FUNCTION "Posizioni Linea" : VOID
TITLE =Gestione posizioni linea pallet
AUTHOR : MassimoZ
FAMILY : NovaSrl
VERSION : 0.1

BEGIN
NETWORK
TITLE ========= Posizioni Zona Accatastatrice 1 =======

NETWORK
TITLE =Pos Fermo pallet indietro *Zona Acc.1*
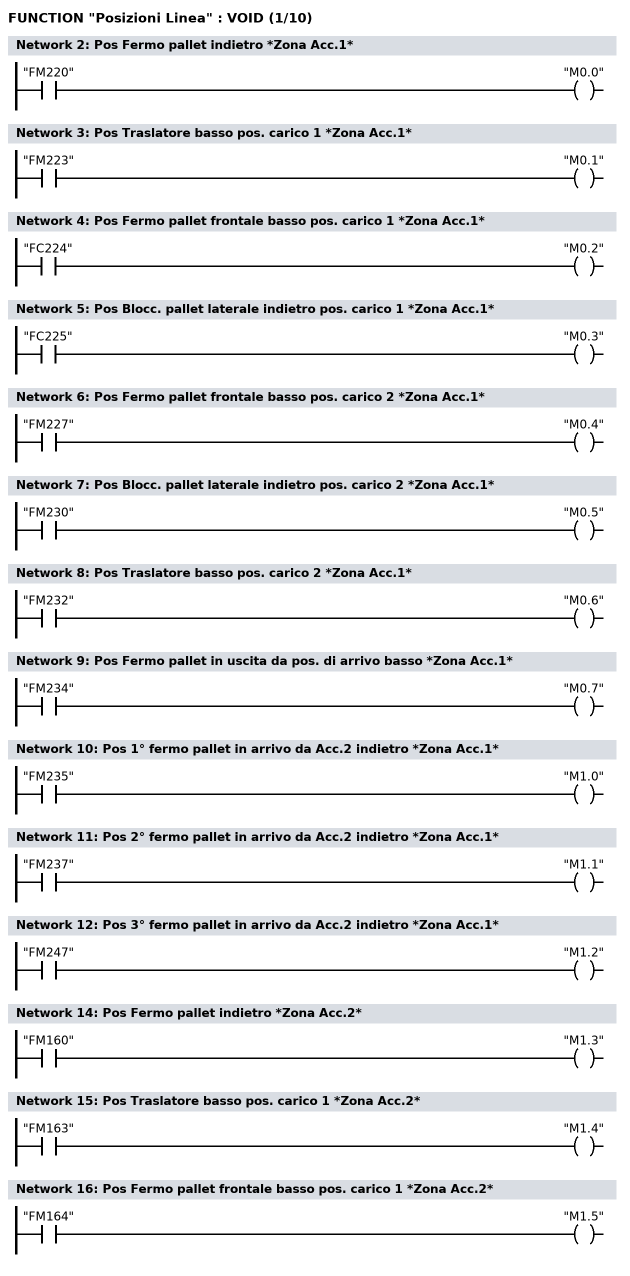
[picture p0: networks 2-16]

      U     "FM220";
      =     "M0.0";
NETWORK
TITLE =Pos Traslatore basso pos. carico 1 *Zona Acc.1*

      U     "FM223";
      =     "M0.1";
NETWORK
TITLE =Pos Fermo pallet frontale basso pos. carico 1 *Zona Acc.1*

      U     "FC224";
      =     "M0.2";
NETWORK
TITLE =Pos Blocc. pallet laterale indietro pos. carico 1 *Zona Acc.1*

      U     "FC225";
      =     "M0.3";
NETWORK
TITLE =Pos Fermo pallet frontale basso pos. carico 2 *Zona Acc.1*

      U     "FM227";
      =     "M0.4";
NETWORK
TITLE =Pos Blocc. pallet laterale indietro pos. carico 2 *Zona Acc.1*

      U     "FM230";
      =     "M0.5";
NETWORK
TITLE =Pos Traslatore basso pos. carico 2 *Zona Acc.1*

      U     "FM232";
      =     "M0.6";
NETWORK
TITLE =Pos Fermo pallet in uscita da pos. di arrivo basso *Zona Acc.1*

      U     "FM234";
      =     "M0.7";
NETWORK
TITLE =Pos 1° fermo pallet in arrivo da Acc.2 indietro *Zona Acc.1*

      U     "FM235";
      =     "M1.0";
NETWORK
TITLE =Pos 2° fermo pallet in arrivo da Acc.2 indietro *Zona Acc.1*

      U     "FM237";
      =     "M1.1";
NETWORK
TITLE =Pos 3° fermo pallet in arrivo da Acc.2 indietro *Zona Acc.1*

      U     "FM247";
      =     "M1.2";
NETWORK
TITLE ========= Posizioni Zona Accatastatrice 2 =======

NETWORK
TITLE =Pos Fermo pallet indietro *Zona Acc.2*

      U     "FM160";
      =     "M1.3";
NETWORK
TITLE =Pos Traslatore basso pos. carico 1 *Zona Acc.2*

      U     "FM163";
      =     "M1.4";
NETWORK
TITLE =Pos Fermo pallet frontale basso pos. carico 1 *Zona Acc.2*

      U     "FM164";
      =     "M1.5";
NETWORK
TITLE =Pos Blocc. pallet laterale indietro pos. carico 1 *Zona Acc.2*
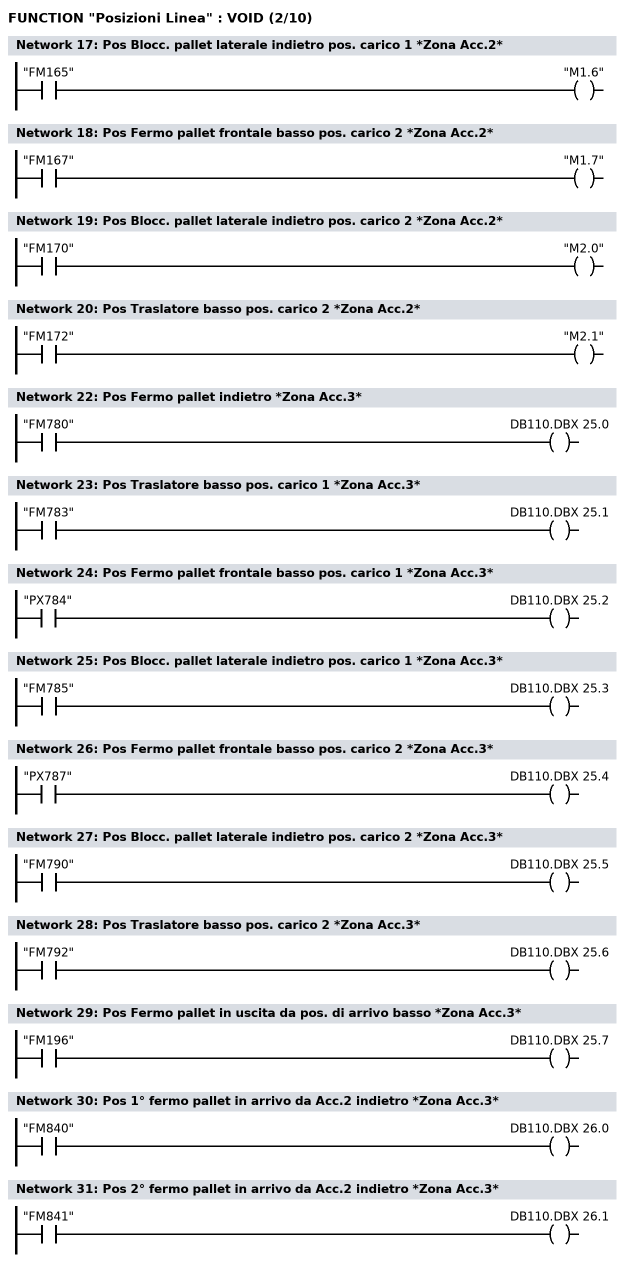
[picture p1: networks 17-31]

      U     "FM165";
      =     "M1.6";
NETWORK
TITLE =Pos Fermo pallet frontale basso pos. carico 2 *Zona Acc.2*

      U     "FM167";
      =     "M1.7";
NETWORK
TITLE =Pos Blocc. pallet laterale indietro pos. carico 2 *Zona Acc.2*

      U     "FM170";
      =     "M2.0";
NETWORK
TITLE =Pos Traslatore basso pos. carico 2 *Zona Acc.2*

      U     "FM172";
      =     "M2.1";
NETWORK
TITLE ========= Posizioni Zona Accatastatrice 3 =======

NETWORK
TITLE =Pos Fermo pallet indietro *Zona Acc.3*

      U     "FM780";
      =     DB110.DBX   25.0;
NETWORK
TITLE =Pos Traslatore basso pos. carico 1 *Zona Acc.3*

      U     "FM783";
      =     DB110.DBX   25.1;
NETWORK
TITLE =Pos Fermo pallet frontale basso pos. carico 1 *Zona Acc.3*

      U     "PX784";
      =     DB110.DBX   25.2;
NETWORK
TITLE =Pos Blocc. pallet laterale indietro pos. carico 1 *Zona Acc.3*

      U     "FM785";
      =     DB110.DBX   25.3;
NETWORK
TITLE =Pos Fermo pallet frontale basso pos. carico 2 *Zona Acc.3*

      U     "PX787";
      =     DB110.DBX   25.4;
NETWORK
TITLE =Pos Blocc. pallet laterale indietro pos. carico 2 *Zona Acc.3*

      U     "FM790";
      =     DB110.DBX   25.5;
NETWORK
TITLE =Pos Traslatore basso pos. carico 2 *Zona Acc.3*

      U     "FM792";
      =     DB110.DBX   25.6;
NETWORK
TITLE =Pos Fermo pallet in uscita da pos. di arrivo basso *Zona Acc.3*

      U     "FM196";
      =     DB110.DBX   25.7;
NETWORK
TITLE =Pos 1° fermo pallet in arrivo da Acc.2 indietro *Zona Acc.3*

      U     "FM840";
      =     DB110.DBX   26.0;
NETWORK
TITLE =Pos 2° fermo pallet in arrivo da Acc.2 indietro *Zona Acc.3*

      U     "FM841";
      =     DB110.DBX   26.1;
NETWORK
TITLE ======== Posizioni Zona Allineamento Bandiere =======

NETWORK
TITLE =Pos Allineamento bandiere alto *Zona Allineamento Bandiere*
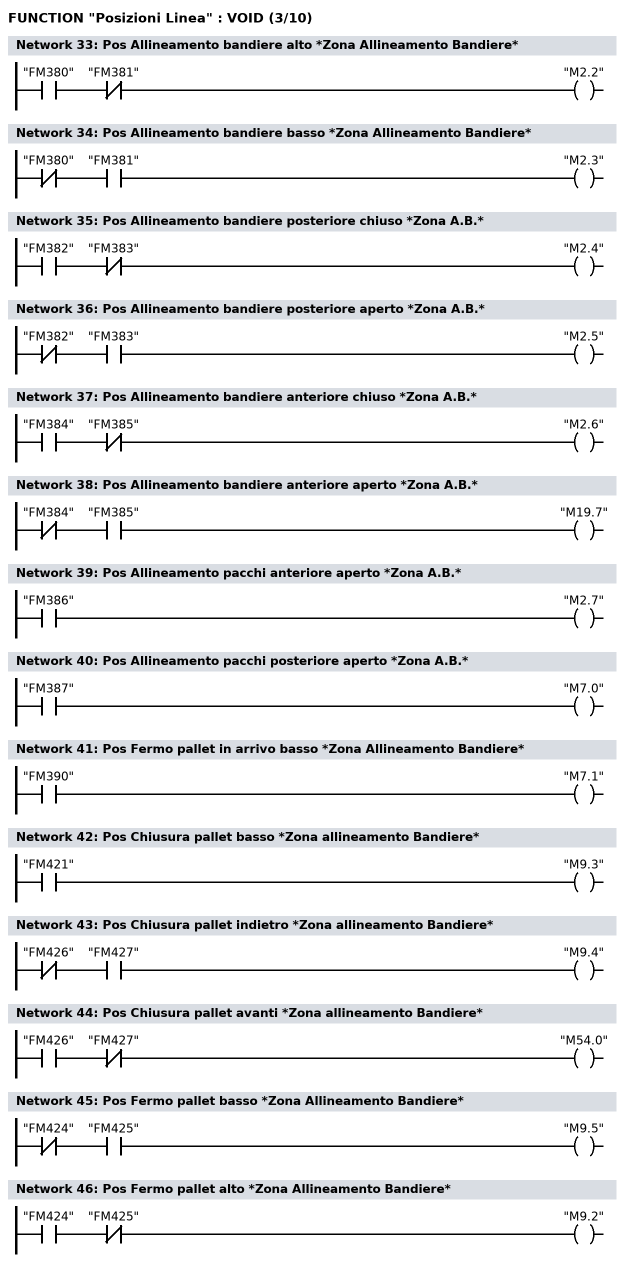
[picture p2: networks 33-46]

      U     "FM380";
      UN    "FM381";
      =     "M2.2";
NETWORK
TITLE =Pos Allineamento bandiere basso *Zona Allineamento Bandiere*

      UN    "FM380";
      U     "FM381";
      =     "M2.3";
NETWORK
TITLE =Pos Allineamento bandiere posteriore chiuso *Zona A.B.*

      U     "FM382";
      UN    "FM383";
      =     "M2.4";
NETWORK
TITLE =Pos Allineamento bandiere posteriore aperto *Zona A.B.*

      UN    "FM382";
      U     "FM383";
      =     "M2.5";
NETWORK
TITLE =Pos Allineamento bandiere anteriore chiuso *Zona A.B.*

      U     "FM384";
      UN    "FM385";
      =     "M2.6";
NETWORK
TITLE =Pos Allineamento bandiere anteriore aperto *Zona A.B.*

      UN    "FM384";
      U     "FM385";
      =     "M19.7";
NETWORK
TITLE =Pos Allineamento pacchi anteriore aperto *Zona A.B.*

      U     "FM386";
      =     "M2.7";
NETWORK
TITLE =Pos Allineamento pacchi posteriore aperto *Zona A.B.*

      U     "FM387";
      =     "M7.0";
NETWORK
TITLE =Pos Fermo pallet in arrivo basso *Zona Allineamento Bandiere*

      U     "FM390";
      =     "M7.1";
NETWORK
TITLE =Pos Chiusura pallet basso *Zona allineamento Bandiere*

      U     "FM421";
      =     "M9.3";
NETWORK
TITLE =Pos Chiusura pallet indietro *Zona allineamento Bandiere*

      UN    "FM426";
      U     "FM427";
      =     "M9.4";
NETWORK
TITLE =Pos Chiusura pallet avanti *Zona allineamento Bandiere*

      U     "FM426";
      UN    "FM427";
      =     "M54.0";
NETWORK
TITLE =Pos Fermo pallet basso *Zona Allineamento Bandiere*

      UN    "FM424";
      U     "FM425";
      =     "M9.5";
NETWORK
TITLE =Pos Fermo pallet alto *Zona Allineamento Bandiere*

      U     "FM424";
      UN    "FM425";
      =     "M9.2";
NETWORK
TITLE ======== Posizioni Zona Piega Bandiere =======

NETWORK
TITLE =Pos Fermo pallet in arrivo basso *Zona Piega Bandiere*
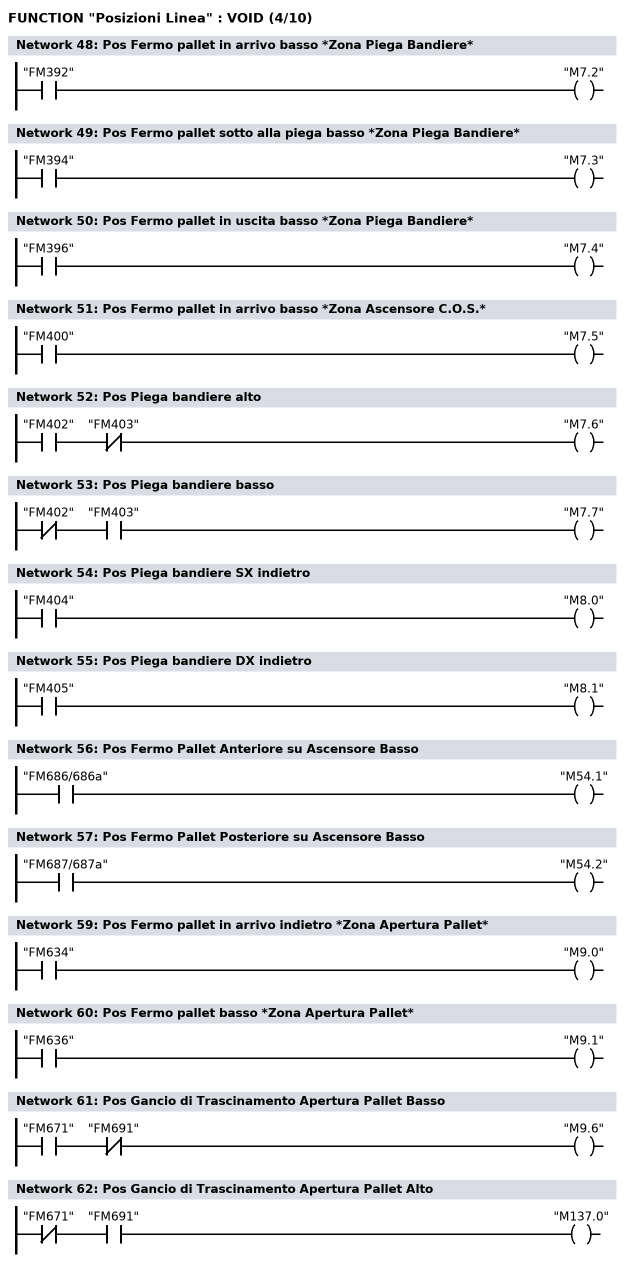
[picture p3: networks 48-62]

      U     "FM392";
      =     "M7.2";
NETWORK
TITLE =Pos Fermo pallet sotto alla piega basso *Zona Piega Bandiere*

      U     "FM394";
      =     "M7.3";
NETWORK
TITLE =Pos Fermo pallet in uscita basso *Zona Piega Bandiere*

      U     "FM396";
      =     "M7.4";
NETWORK
TITLE =Pos Fermo pallet in arrivo basso *Zona Ascensore C.O.S.*

      U     "FM400";
      =     "M7.5";
NETWORK
TITLE =Pos Piega bandiere alto

      U     "FM402";
      UN    "FM403";
      =     "M7.6";
NETWORK
TITLE =Pos Piega bandiere basso

      UN    "FM402";
      U     "FM403";
      =     "M7.7";
NETWORK
TITLE =Pos Piega bandiere SX indietro

      U     "FM404";
      =     "M8.0";
NETWORK
TITLE =Pos Piega bandiere DX indietro

      U     "FM405";
      =     "M8.1";
NETWORK
TITLE =Pos Fermo Pallet Anteriore su Ascensore Basso

      U     "FM686/686a";
      =     "M54.1";
NETWORK
TITLE =Pos Fermo Pallet Posteriore su Ascensore Basso

      U     "FM687/687a";
      =     "M54.2";
NETWORK
TITLE ======== Posizioni Zona Apertura Pallet =======

NETWORK
TITLE =Pos Fermo pallet in arrivo indietro *Zona Apertura Pallet*

      U     "FM634";
      =     "M9.0";
NETWORK
TITLE =Pos Fermo pallet basso *Zona Apertura Pallet*

      U     "FM636";
      =     "M9.1";
NETWORK
TITLE =Pos Gancio di Trascinamento Apertura Pallet Basso

      U     "FM671";
      UN    "FM691";
      =     "M9.6";
NETWORK
TITLE =Pos Gancio di Trascinamento Apertura Pallet Alto

      UN    "FM671";
      U     "FM691";
      =     "M137.0";
NETWORK
TITLE =Pos Dente apertura pallet basso *Zona Apertura Pallet*
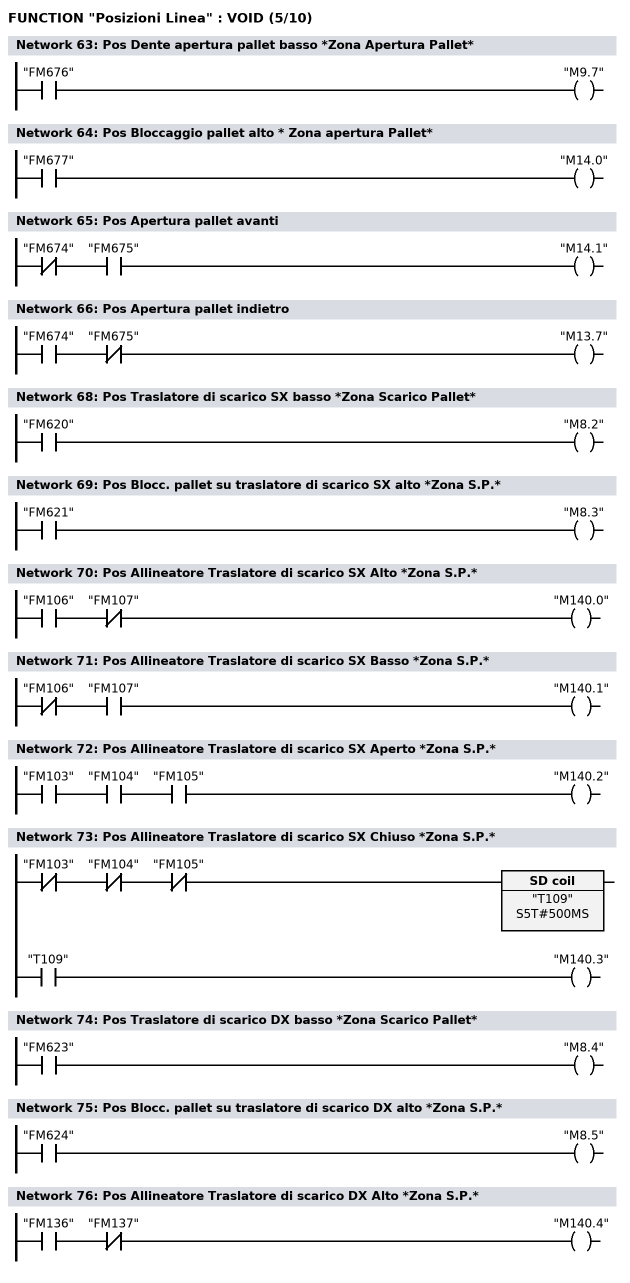
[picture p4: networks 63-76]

      U     "FM676";
      =     "M9.7";
NETWORK
TITLE =Pos Bloccaggio pallet alto * Zona apertura Pallet*

      U     "FM677";
      =     "M14.0";
NETWORK
TITLE =Pos Apertura pallet avanti

      UN    "FM674";
      U     "FM675";
      =     "M14.1";
NETWORK
TITLE =Pos Apertura pallet indietro

      U     "FM674";
      UN    "FM675";
      =     "M13.7";
NETWORK
TITLE ======== Posizioni Zona Scarico Pallet =======

NETWORK
TITLE =Pos Traslatore di scarico SX basso *Zona Scarico Pallet*

      U     "FM620";
      =     "M8.2";
NETWORK
TITLE =Pos Blocc. pallet su traslatore di scarico SX alto *Zona S.P.*

      U     "FM621";
      =     "M8.3";
NETWORK
TITLE =Pos Allineatore Traslatore di scarico SX Alto *Zona S.P.*

      U     "FM106";
      UN    "FM107";
      =     "M140.0";
NETWORK
TITLE =Pos Allineatore Traslatore di scarico SX Basso *Zona S.P.*

      UN    "FM106";
      U     "FM107";
      =     "M140.1";
NETWORK
TITLE =Pos Allineatore Traslatore di scarico SX Aperto *Zona S.P.*

      U     "FM103";
      U     "FM104";
      U     "FM105";
      =     "M140.2";
NETWORK
TITLE =Pos Allineatore Traslatore di scarico SX Chiuso *Zona S.P.*

      UN    "FM103";
      UN    "FM104";
      UN    "FM105";
      L     S5T#500MS;
      SE    "T109";
      NOP   0;
      NOP   0;
      NOP   0;
      U     "T109";
      =     "M140.3";
NETWORK
TITLE =Pos Traslatore di scarico DX basso *Zona Scarico Pallet*

      U     "FM623";
      =     "M8.4";
NETWORK
TITLE =Pos Blocc. pallet su traslatore di scarico DX alto *Zona S.P.*

      U     "FM624";
      =     "M8.5";
NETWORK
TITLE =Pos Allineatore Traslatore di scarico DX Alto *Zona S.P.*

      U     "FM136";
      UN    "FM137";
      =     "M140.4";
NETWORK
TITLE =Pos Allineatore Traslatore di scarico DX Basso *Zona S.P.*
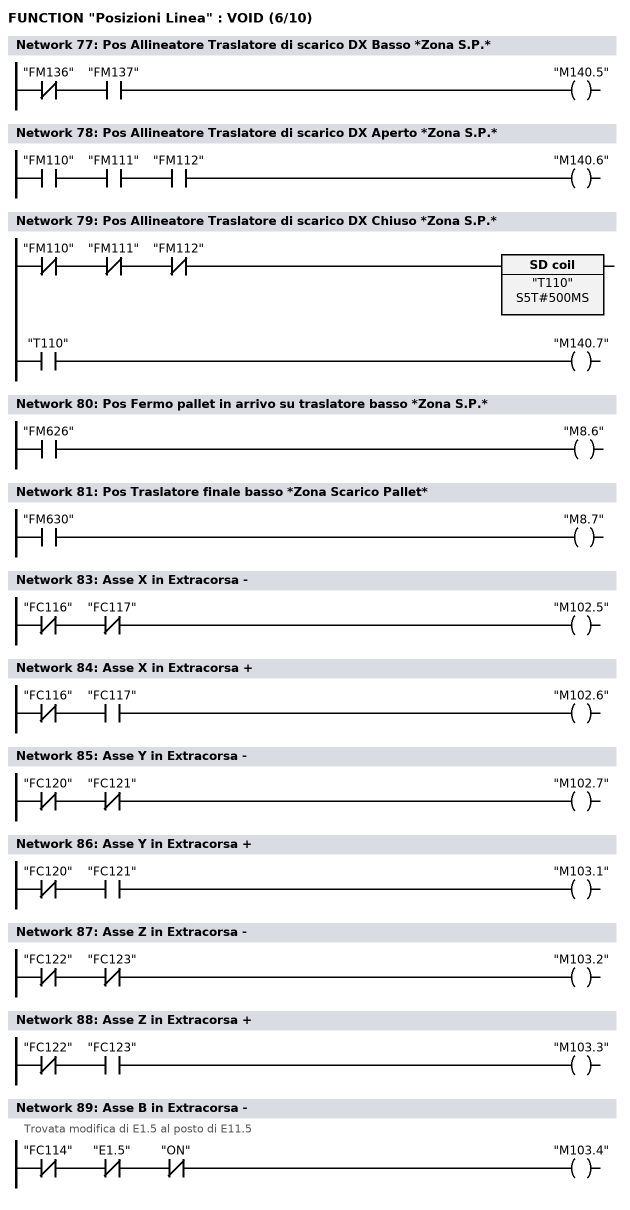
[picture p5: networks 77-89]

      UN    "FM136";
      U     "FM137";
      =     "M140.5";
NETWORK
TITLE =Pos Allineatore Traslatore di scarico DX Aperto *Zona S.P.*

      U     "FM110";
      U     "FM111";
      U     "FM112";
      =     "M140.6";
NETWORK
TITLE =Pos Allineatore Traslatore di scarico DX Chiuso *Zona S.P.*

      UN    "FM110";
      UN    "FM111";
      UN    "FM112";
      L     S5T#500MS;
      SE    "T110";
      NOP   0;
      NOP   0;
      NOP   0;
      U     "T110";
      =     "M140.7";
NETWORK
TITLE =Pos Fermo pallet in arrivo su traslatore basso *Zona S.P.*

      U     "FM626";
      =     "M8.6";
NETWORK
TITLE =Pos Traslatore finale basso *Zona Scarico Pallet*

      U     "FM630";
      =     "M8.7";
NETWORK
TITLE ======== Posizioni Boxing ======

NETWORK
TITLE =Asse X in Extracorsa -

      UN    "FC116";
      UN    "FC117";
      =     "M102.5";
NETWORK
TITLE =Asse X in Extracorsa +

      UN    "FC116";
      U     "FC117";
      =     "M102.6";
NETWORK
TITLE =Asse Y in Extracorsa -

      UN    "FC120";
      UN    "FC121";
      =     "M102.7";
NETWORK
TITLE =Asse Y in Extracorsa +

      UN    "FC120";
      U     "FC121";
      =     "M103.1";
NETWORK
TITLE =Asse Z in Extracorsa -

      UN    "FC122";
      UN    "FC123";
      =     "M103.2";
NETWORK
TITLE =Asse Z in Extracorsa +

      UN    "FC122";
      U     "FC123";
      =     "M103.3";
NETWORK
TITLE =Asse B in Extracorsa -
//Trovata modifica di E1.5 al posto di E11.5
      UN    "FC114";
      UN    "E1.5";
      UN    "ON";
      =     "M103.4";
NETWORK
TITLE =Asse B in Extracorsa +
//Trovata modifica di E1.5 al posto di E11.5
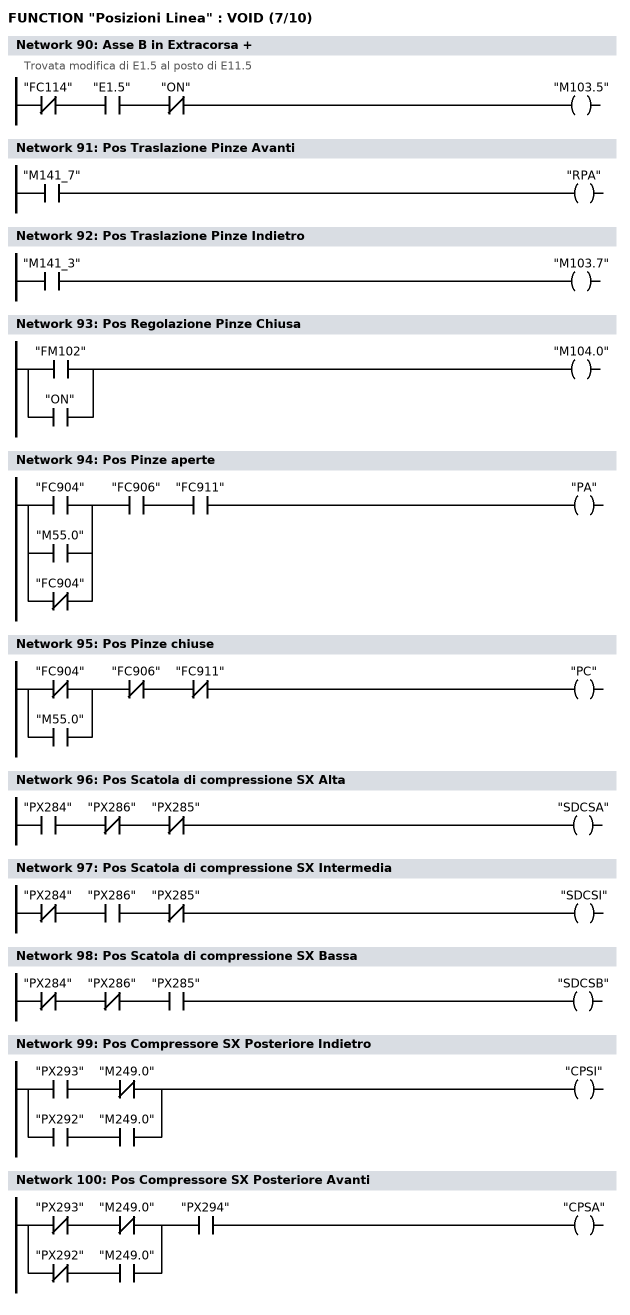
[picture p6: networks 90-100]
      UN    "FC114";
      U     "E1.5";
      UN    "ON";
      =     "M103.5";
NETWORK
TITLE =Pos Traslazione Pinze Avanti

      U     "M141_7";
      =     "RPA";
NETWORK
TITLE =Pos Traslazione Pinze Indietro

      U     "M141_3";
      =     "M103.7";
NETWORK
TITLE =Pos Regolazione Pinze Chiusa

      O     "FM102";
      O     "ON";
      =     "M104.0";
NETWORK
TITLE =Pos Pinze aperte

      U(    ;
      O     "FC904";
      O     "M55.0";
      ON    "FC904";
      )     ;
      U     "FC906";
      U     "FC911";
      =     "PA";
NETWORK
TITLE =Pos Pinze chiuse

      U(    ;
      ON    "FC904";
      O     "M55.0";
      )     ;
      UN    "FC906";
      UN    "FC911";
      =     "PC";
NETWORK
TITLE =Pos Scatola di compressione SX Alta

      U     "PX284";
      UN    "PX286";
      UN    "PX285";
      =     "SDCSA";
NETWORK
TITLE =Pos Scatola di compressione SX Intermedia

      UN    "PX284";
      U     "PX286";
      UN    "PX285";
      =     "SDCSI";
NETWORK
TITLE =Pos Scatola di compressione SX Bassa

      UN    "PX284";
      UN    "PX286";
      U     "PX285";
      =     "SDCSB";
NETWORK
TITLE =Pos Compressore SX Posteriore Indietro

      U     "PX293";
      UN    "M249.0";
      O     ;
      U     "PX292";
      U     "M249.0";
      =     "CPSI";
NETWORK
TITLE =Pos Compressore SX Posteriore Avanti

      U(    ;
      UN    "PX293";
      UN    "M249.0";
      O     ;
      UN    "PX292";
      U     "M249.0";
      )     ;
      U     "PX294";
      =     "CPSA";
NETWORK
TITLE =Pos Compressore SX Laterale Indietro
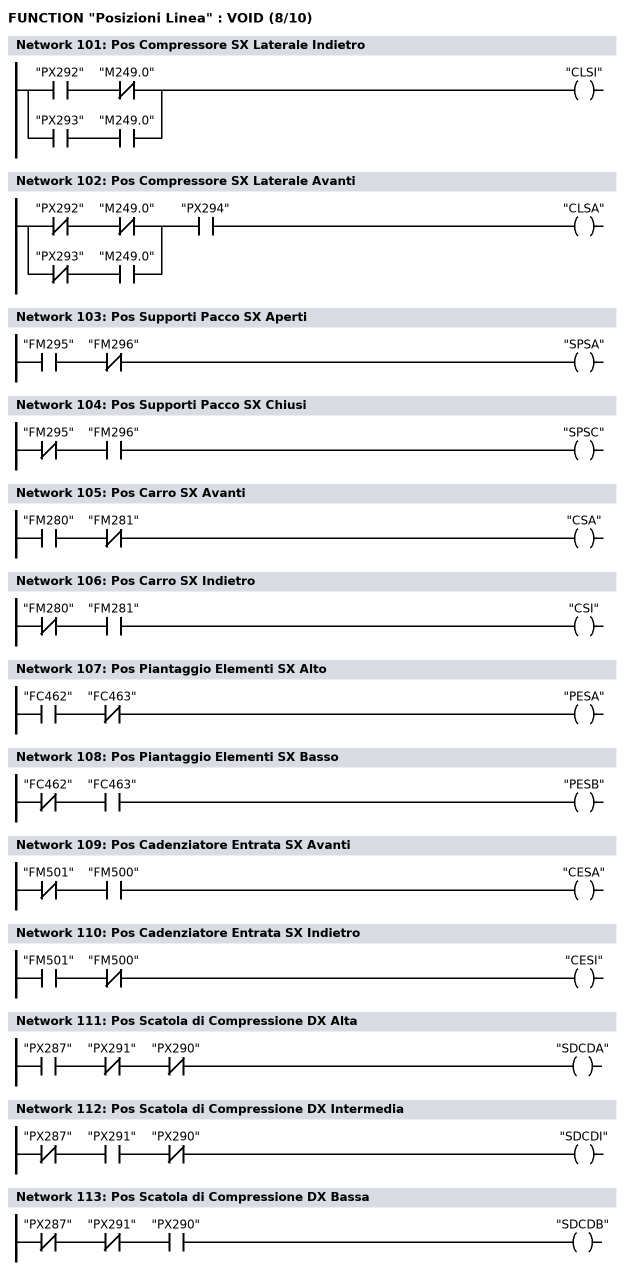
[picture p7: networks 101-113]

      U     "PX292";
      UN    "M249.0";
      O     ;
      U     "PX293";
      U     "M249.0";
      =     "CLSI";
NETWORK
TITLE =Pos Compressore SX Laterale Avanti

      U(    ;
      UN    "PX292";
      UN    "M249.0";
      O     ;
      UN    "PX293";
      U     "M249.0";
      )     ;
      U     "PX294";
      =     "CLSA";
NETWORK
TITLE =Pos Supporti Pacco SX Aperti

      U     "FM295";
      UN    "FM296";
      =     "SPSA";
NETWORK
TITLE =Pos Supporti Pacco SX Chiusi

      UN    "FM295";
      U     "FM296";
      =     "SPSC";
NETWORK
TITLE =Pos Carro SX Avanti

      U     "FM280";
      UN    "FM281";
      =     "CSA";
NETWORK
TITLE =Pos Carro SX Indietro

      UN    "FM280";
      U     "FM281";
      =     "CSI";
NETWORK
TITLE =Pos Piantaggio Elementi SX Alto

      U     "FC462";
      UN    "FC463";
      =     "PESA";
NETWORK
TITLE =Pos Piantaggio Elementi SX Basso

      UN    "FC462";
      U     "FC463";
      =     "PESB";
NETWORK
TITLE =Pos Cadenziatore Entrata SX Avanti

      UN    "FM501";
      U     "FM500";
      =     "CESA";
NETWORK
TITLE =Pos Cadenziatore Entrata SX Indietro

      U     "FM501";
      UN    "FM500";
      =     "CESI";
NETWORK
TITLE =Pos Scatola di Compressione DX Alta

      U     "PX287";
      UN    "PX291";
      UN    "PX290";
      =     "SDCDA";
NETWORK
TITLE =Pos Scatola di Compressione DX Intermedia

      UN    "PX287";
      U     "PX291";
      UN    "PX290";
      =     "SDCDI";
NETWORK
TITLE =Pos Scatola di Compressione DX Bassa

      UN    "PX287";
      UN    "PX291";
      U     "PX290";
      =     "SDCDB";
NETWORK
TITLE =Pos Compressore Posteriore DX Indietro
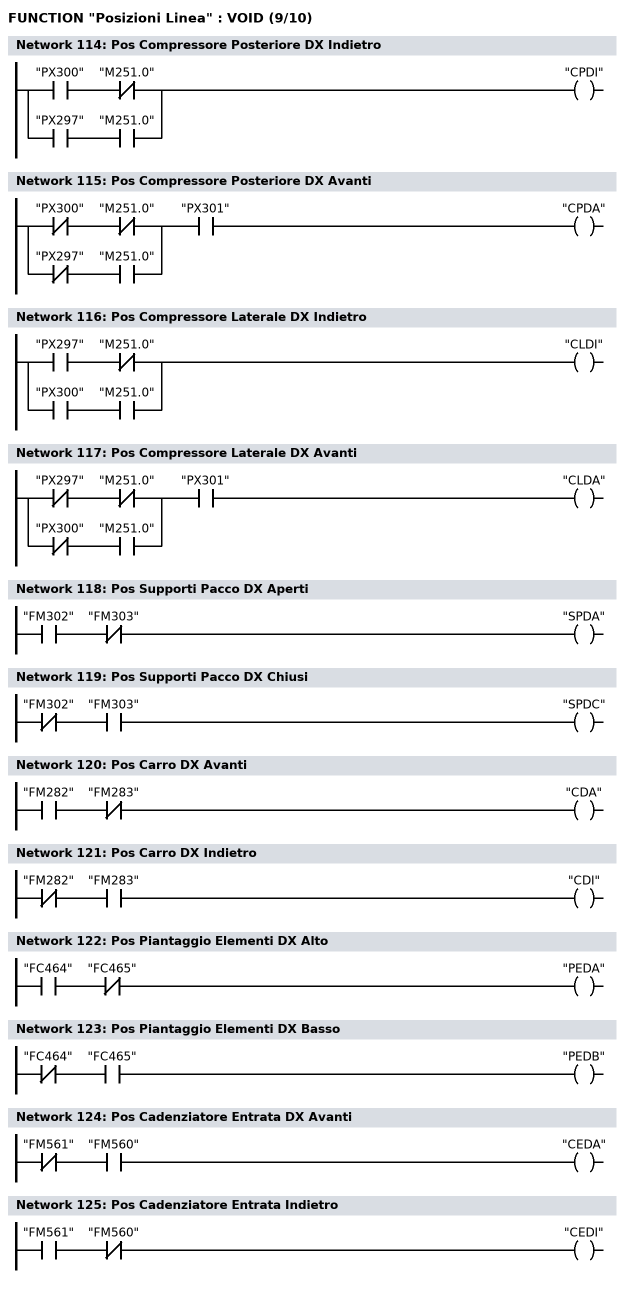
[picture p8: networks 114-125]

      U     "PX300";
      UN    "M251.0";
      O     ;
      U     "PX297";
      U     "M251.0";
      =     "CPDI";
NETWORK
TITLE =Pos Compressore Posteriore DX Avanti

      U(    ;
      UN    "PX300";
      UN    "M251.0";
      O     ;
      UN    "PX297";
      U     "M251.0";
      )     ;
      U     "PX301";
      =     "CPDA";
NETWORK
TITLE =Pos Compressore Laterale DX Indietro

      U     "PX297";
      UN    "M251.0";
      O     ;
      U     "PX300";
      U     "M251.0";
      =     "CLDI";
NETWORK
TITLE =Pos Compressore Laterale DX Avanti

      U(    ;
      UN    "PX297";
      UN    "M251.0";
      O     ;
      UN    "PX300";
      U     "M251.0";
      )     ;
      U     "PX301";
      =     "CLDA";
NETWORK
TITLE =Pos Supporti Pacco DX Aperti

      U     "FM302";
      UN    "FM303";
      =     "SPDA";
NETWORK
TITLE =Pos Supporti Pacco DX Chiusi

      UN    "FM302";
      U     "FM303";
      =     "SPDC";
NETWORK
TITLE =Pos Carro DX Avanti

      U     "FM282";
      UN    "FM283";
      =     "CDA";
NETWORK
TITLE =Pos Carro DX Indietro

      UN    "FM282";
      U     "FM283";
      =     "CDI";
NETWORK
TITLE =Pos Piantaggio Elementi DX Alto

      U     "FC464";
      UN    "FC465";
      =     "PEDA";
NETWORK
TITLE =Pos Piantaggio Elementi DX Basso

      UN    "FC464";
      U     "FC465";
      =     "PEDB";
NETWORK
TITLE =Pos Cadenziatore Entrata DX Avanti

      UN    "FM561";
      U     "FM560";
      =     "CEDA";
NETWORK
TITLE =Pos Cadenziatore Entrata Indietro

      U     "FM561";
      UN    "FM560";
      =     "CEDI";
NETWORK
TITLE =Pos Braccio di Spostamento da Nastro1 a Nastro2 Avanti
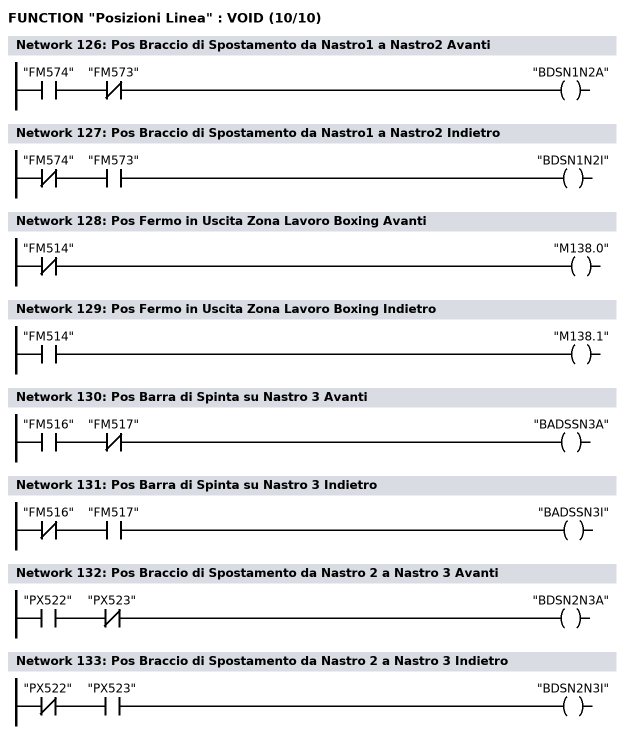
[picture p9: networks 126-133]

      U     "FM574";
      UN    "FM573";
      =     "BDSN1N2A";
NETWORK
TITLE =Pos Braccio di Spostamento da Nastro1 a Nastro2 Indietro

      UN    "FM574";
      U     "FM573";
      =     "BDSN1N2I";
NETWORK
TITLE =Pos Fermo in Uscita Zona Lavoro Boxing Avanti

      UN    "FM514";
      =     "M138.0";
NETWORK
TITLE =Pos Fermo in Uscita Zona Lavoro Boxing Indietro

      U     "FM514";
      =     "M138.1";
NETWORK
TITLE =Pos Barra di Spinta su Nastro 3 Avanti

      U     "FM516";
      UN    "FM517";
      =     "BADSSN3A";
NETWORK
TITLE =Pos Barra di Spinta su Nastro 3 Indietro

      UN    "FM516";
      U     "FM517";
      =     "BADSSN3I";
NETWORK
TITLE =Pos Braccio di Spostamento da Nastro 2 a Nastro 3 Avanti

      U     "PX522";
      UN    "PX523";
      =     "BDSN2N3A";
NETWORK
TITLE =Pos Braccio di Spostamento da Nastro 2 a Nastro 3 Indietro

      UN    "PX522";
      U     "PX523";
      =     "BDSN2N3I";
END_FUNCTION

